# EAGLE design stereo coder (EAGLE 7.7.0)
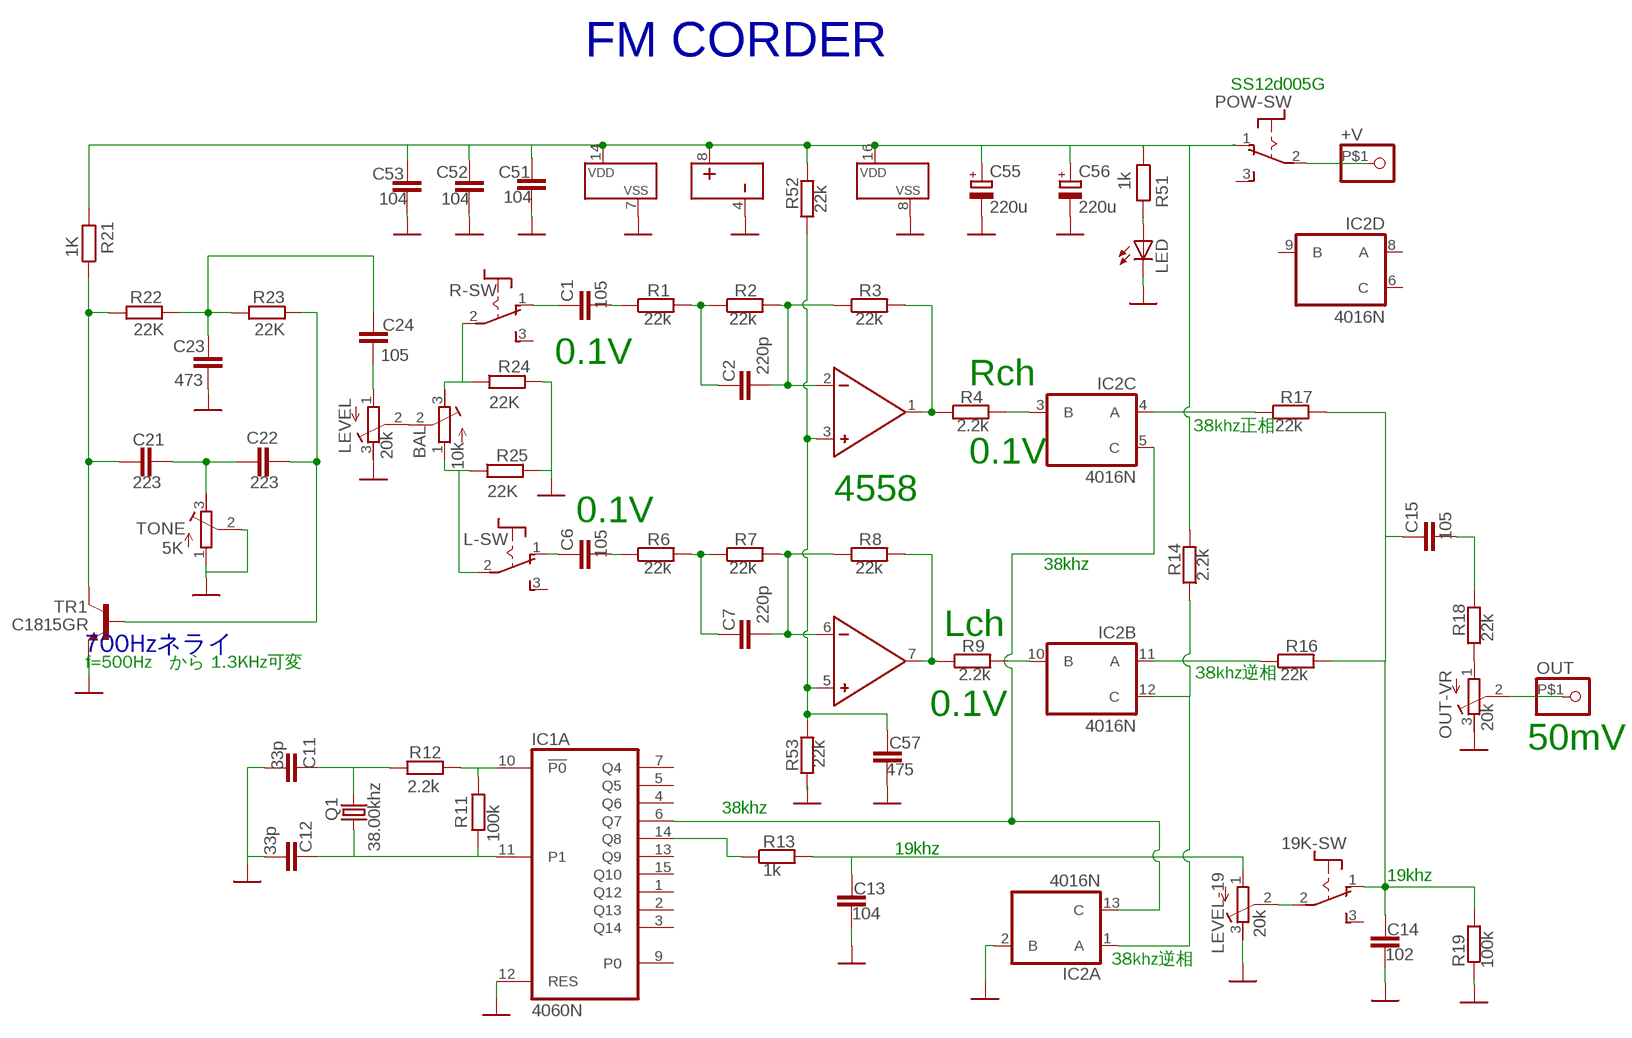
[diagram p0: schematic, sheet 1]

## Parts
19K-SW  POW-SW  [POW-SW]
+V  PINHD-1X1  [1X01]
BAL  10k  R-TRIMM3296W  [RTRIM3296W]
C1  105  C-EU050-024X044  [C050-024X044]
C2  220p  C-EU050-024X044  [C050-024X044]
C6  105  C-EU050-024X044  [C050-024X044]
C7  220p  C-EU050-024X044  [C050-024X044]
C11  33p  C-EU050-024X044  [C050-024X044]
C12  33p  C-EU050-024X044  [C050-024X044]
C13  104  C-EU050-024X044  [C050-024X044]
C14  102  C-EU050-024X044  [C050-024X044]
C15  105  C-EU050-024X044  [C050-024X044]
C21  223  C-EU050-024X044  [C050-024X044]
C22  223  C-EU050-024X044  [C050-024X044]
C23  473  C-EU050-024X044  [C050-024X044]
C24  105  C-EU050-024X044  [C050-024X044]
C51  104  C-EU050-024X044  [C050-024X044]
C52  104  C-EU050-024X044  [C050-024X044]
C53  104  C-EU050-024X044  [C050-024X044]
C55  220u  CPOL-EUE2.5-7  [E2,5-7]
C56  220u  CPOL-EUE2.5-7  [E2,5-7]
C57  475  C-EU050-024X044  [C050-024X044]
IC1  4060N  [DIL16]
IC2  4016N  [DIL14]
L-SW  POW-SW  [POW-SW]
LED  LEDIRL80A  [IRL80A]
LEVEL  20k  R-TRIMM3296W  [RTRIM3296W]
LEVEL-19  20k  R-TRIMM3296W  [RTRIM3296W]
OUT  PINHD-1X1  [1X01]
OUT-VR  20k  R-TRIMM3296W  [RTRIM3296W]
Q1  38.00khz  CRYSTALTC38H  [TC38H]
R1  22k  R-EU_0204/5  [0204/5]
R2  22k  R-EU_0204/5  [0204/5]
R3  22k  R-EU_0204/5  [0204/5]
R4  2.2k  R-EU_0204/5  [0204/5]
R6  22k  R-EU_0204/5  [0204/5]
R7  22k  R-EU_0204/5  [0204/5]
R8  22k  R-EU_0204/5  [0204/5]
R9  2.2k  R-EU_0204/5  [0204/5]
R11  100k  R-EU_0204/5  [0204/5]
R12  2.2k  R-EU_0204/5  [0204/5]
R13  1k  R-EU_0204/5  [0204/5]
R14  2.2k  R-EU_0204/5  [0204/5]
R16  22k  R-EU_0204/5  [0204/5]
R17  22k  R-EU_0204/5  [0204/5]
R18  22k  R-EU_0204/5  [0204/5]
R19  100k  R-EU_0204/5  [0204/5]
R21  1K  R-EU_0204/5  [0204/5]
R22  22K  R-EU_0204/5  [0204/5]
R23  22K  R-EU_0204/5  [0204/5]
R24  22K  R-EU_0204/5  [0204/5]
R25  22K  R-EU_0204/5  [0204/5]
R51  1k  R-EU_0204/5  [0204/5]
R52  22k  R-EU_0204/5  [0204/5]
R53  22k  R-EU_0204/5  [0204/5]
R-SW  POW-SW  [POW-SW]
TONE  5K  R-TRIMM3296W  [RTRIM3296W]
TR1  C1815GR  2SC1815L  [TO92-1815]
U$1  4558  [DIL08]
U$3  POW-SW  [POW-SW]

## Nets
+V: C51.1 C52.1 C53.1 C55.+ C56.+ IC1.16(P:VDD) IC2.14(P:VDD) R14.2 R21.2 R51.1 R52.2 U$1.8 U$3.1(O)
GND: C11.2 C12.2 C13.2 C14.2 C23.2 C51.2 C52.2 C53.2 C55.- C56.- C57.2 IC1.8(P:VSS) IC1.12(A:RES) IC2.2(A:B) IC2.7(P:VSS) LED.K(C) LEVEL-19.3(A) LEVEL.3(A) OUT-VR.3(A) R19.2 R24.2 R25.2 R53.1 TONE.1(E) TONE.2(S) TR1.E U$1.4
N$1: C2.1 R1.2 R2.1
N$2: C2.2 R2.2 R3.1 U$1.2
N$3: R3.2 R4.1 U$1.1
N$4: C1.2 R1.1
N$5: C1.1 R-SW.1(O)
N$6: C7.1 R6.2 R7.1
N$7: C7.2 R7.2 R8.1 U$1.6
N$8: R8.2 R9.1 U$1.7
N$9: C6.2 R6.1
N$10: C6.1 L-SW.1(O)
N$11: IC1.14(A:Q8) R13.1
N$13: IC2.3(C:B) R4.2
N$14: IC2.10(B:B) R9.2
N$15: IC2.4(C:A) R17.1
N$16: IC2.11(B:A) R16.1
N$17: 19K-SW.1(O) C14.1 C15.1 R16.2 R17.2 R19.1
N$18: +V.P$1 U$3.2(P)
N$19: IC1.6(A:Q7) IC2.5(C:C) IC2.13(A:C)
N$20: IC1.10(A:!P0) R11.1 R12.1
N$21: C12.1 IC1.11(A:P1) Q1.1 R11.2
N$22: C11.1 Q1.2 R12.2
N$23: C21.1 C22.2 TONE.3(A)
N$24: IC2.1(A:A) IC2.12(B:C) R14.1
N$25: C13.1 LEVEL-19.1(E) R13.2
N$26: C15.2 R18.2
N$27: C22.1 R23.2 TR1.B
N$28: C21.2 R21.1 R22.1 TR1.C
N$29: BAL.2(S) LEVEL.2(S)
N$30: LED.A R51.2
N$31: OUT-VR.1(E) R18.1
N$32: OUT-VR.2(S) OUT.P$1
N$33: 19K-SW.2(P) LEVEL-19.2(S)
N$34: C57.1 R52.1 R53.2 U$1.3 U$1.5
N$52: C23.1 C24.1 R22.2 R23.1
N$53: C24.2 LEVEL.1(E)
N$54: BAL.3(A) R24.1 R-SW.2(P)
N$55: BAL.1(E) L-SW.2(P) R25.1
Unconnected: 19K-SW.3(S) IC1.1(A:Q12) IC1.2(A:Q13) IC1.3(A:Q14) IC1.4(A:Q6) IC1.5(A:Q5) IC1.7(A:Q4) IC1.9(A:P0) IC1.13(A:Q9) IC1.15(A:Q10) IC2.6(D:C) IC2.8(D:A) IC2.9(D:B) L-SW.3(S) R-SW.3(S) U$3.3(S)

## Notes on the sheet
- FM CORDER
- SS12d005G
- 0.1V
- Rch
- 38khz正相
- 0.1V
- 4558
- 0.1V
- 38khz
- Lch
- 700Hzネライ
- f=500Hz　から 1.3KHz可変
- 38khz逆相
- 0.1V
- 50mV
- 38khz
- 19khz
- 19khz
- 38khz逆相

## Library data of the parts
19K-SW L-SW R-SW U$3 = switch:POW-SW
+V OUT = pinhead:PINHD-1X1: PIN HEADER
BAL LEVEL LEVEL-19 OUT-VR TONE = resistor:R-TRIMM: Trimm resistor
C1 C2 C6 C7 C11-C15 C21-C24 C51-C53 C57 = resistor:C-EU: CAPACITOR, European symbol
C55 C56 = resistor:CPOL-EU: POLARIZED CAPACITOR, European symbol
IC1 = 40xx:4060: 14-stage binary/ripple COUNTER
IC2 = 40xx:4016: Quad bilateral ANALOG SWITCH
LED = led:LED: LED
Q1 = crystal:CRYSTAL: CRYSTAL; OC_FARNELL: unknown; OC_NEWARK: unknown
R1-R4 R6-R9 R11-R14 R16-R19 R21-R25 R51-R53 = resistor:R-EU_: RESISTOR, European symbol
TR1 = transistor:2SC1815L
U$1 = ic-package:4558

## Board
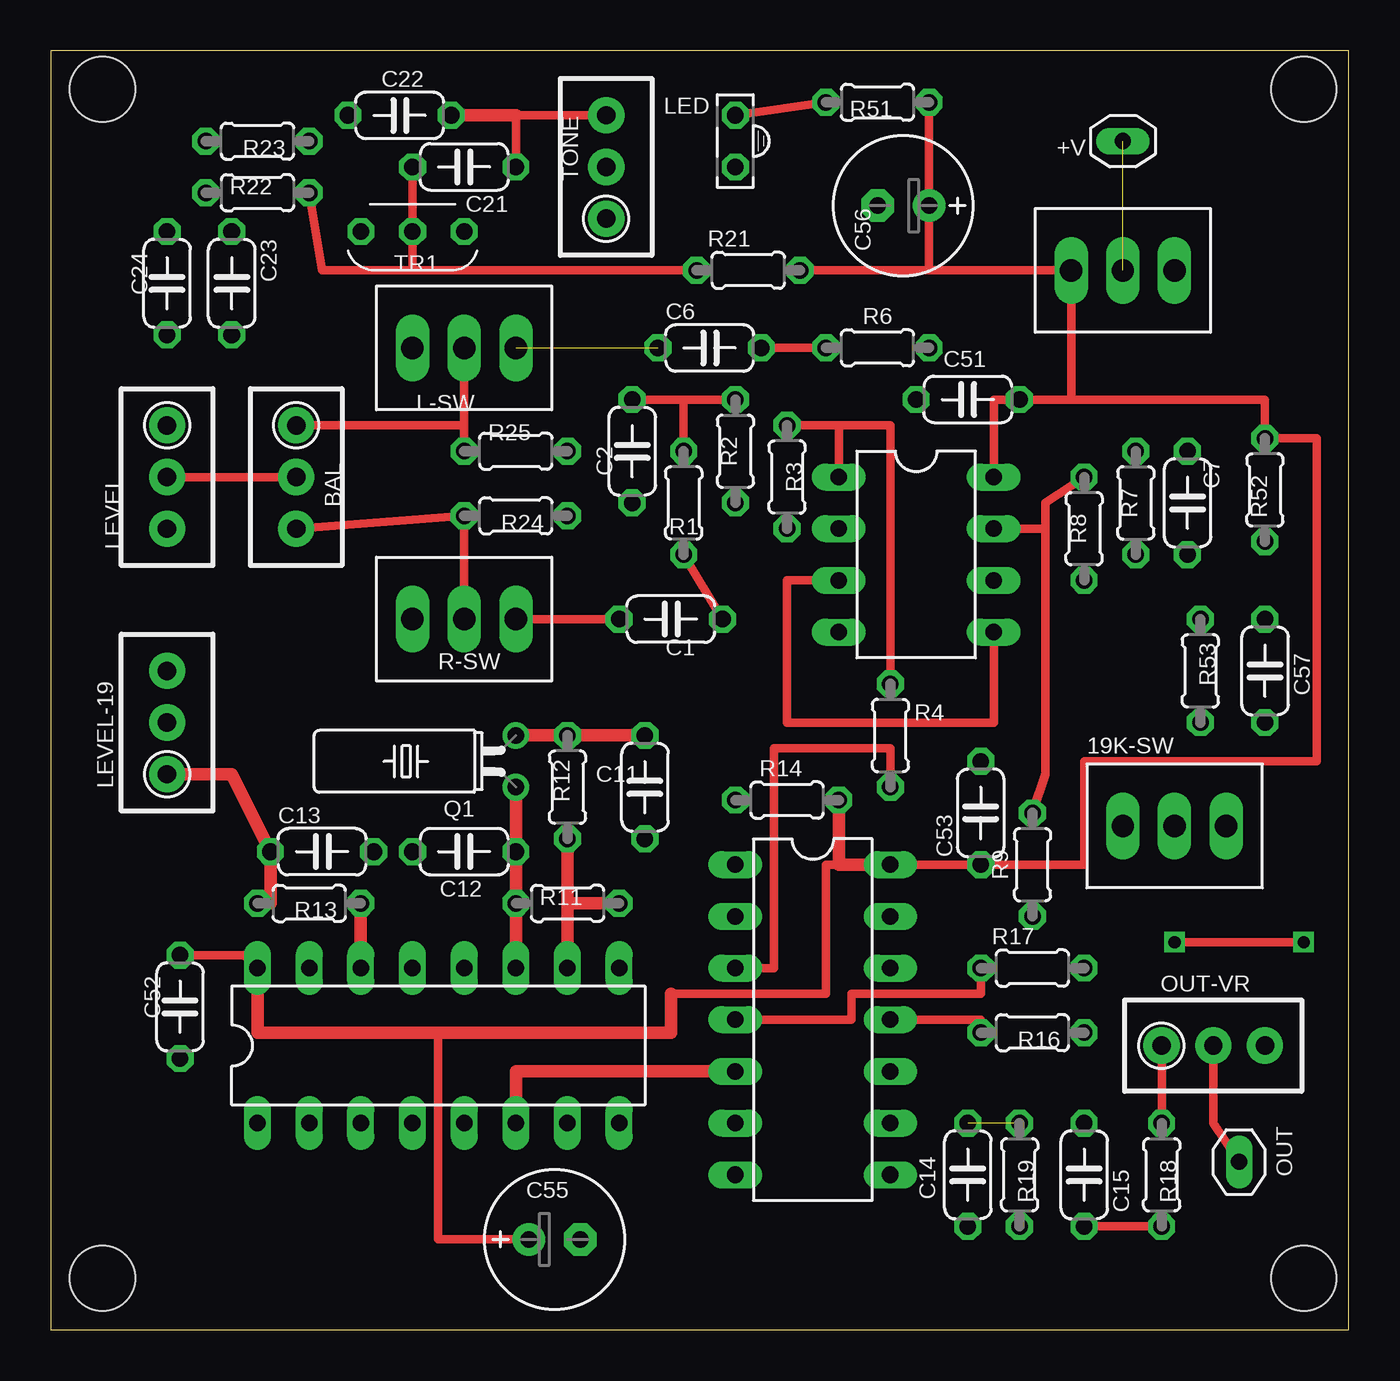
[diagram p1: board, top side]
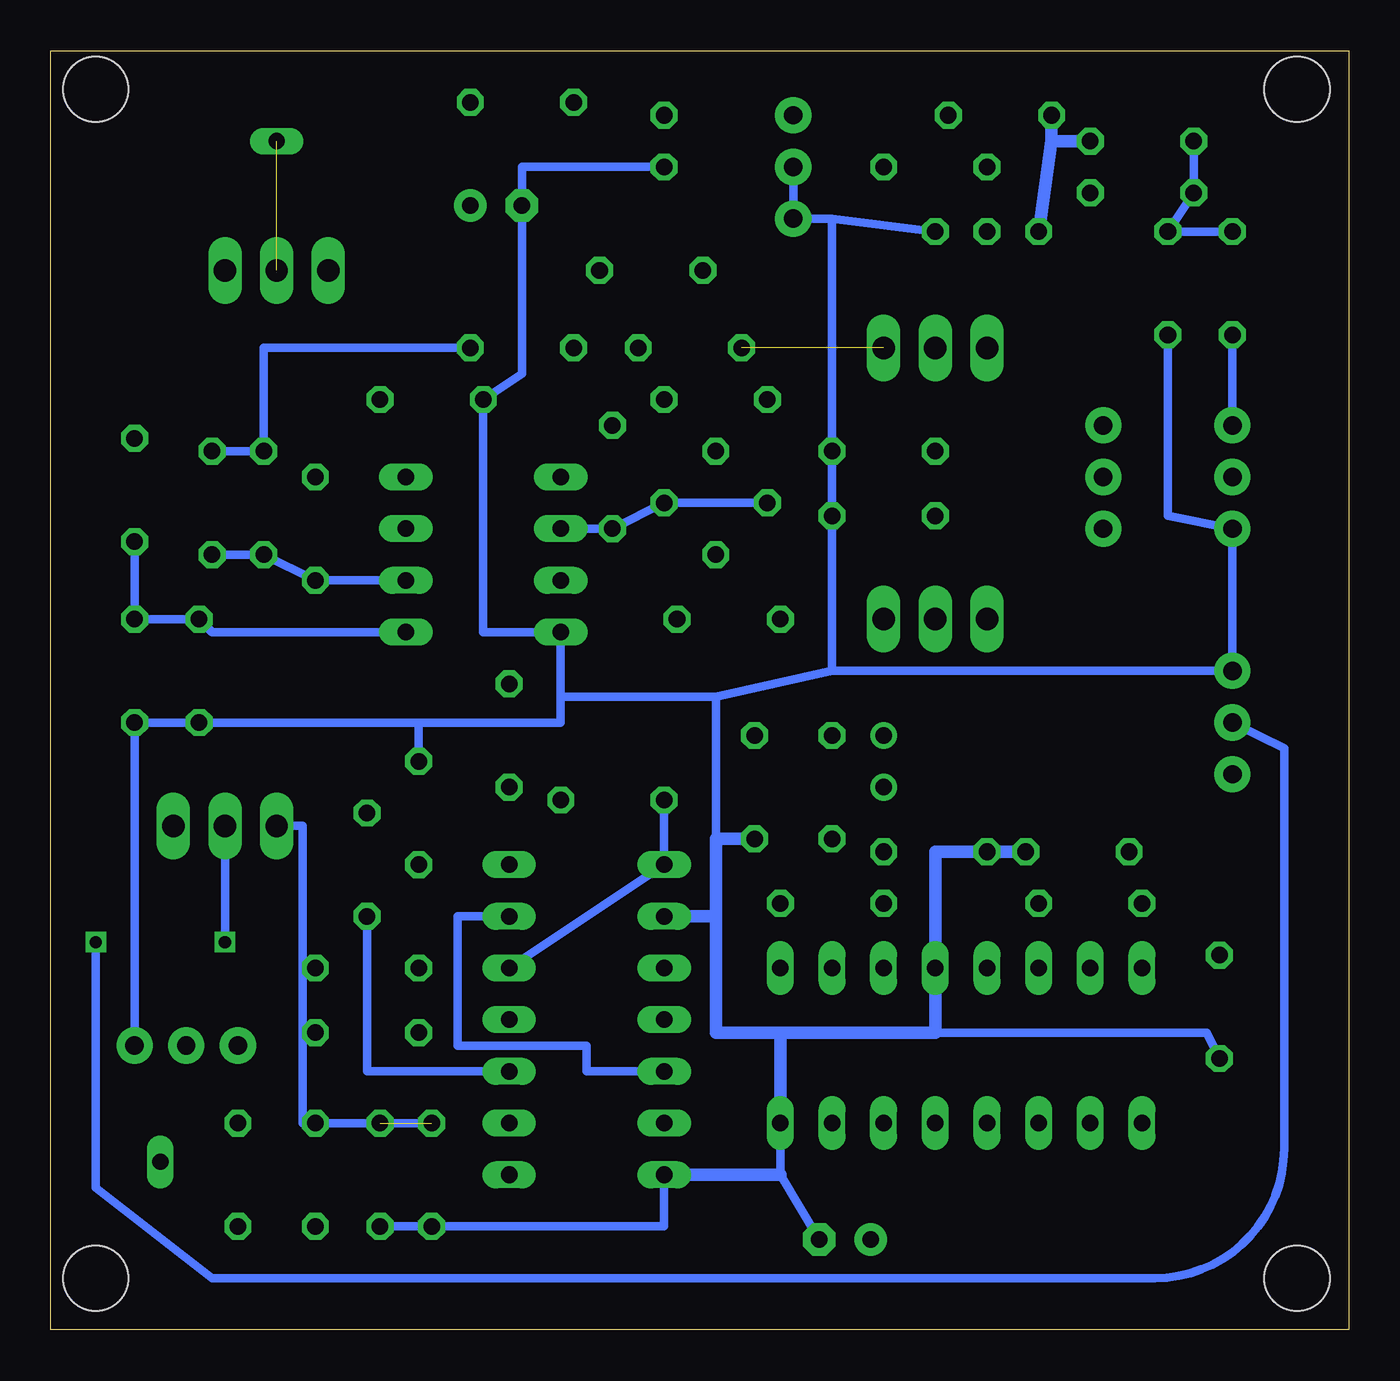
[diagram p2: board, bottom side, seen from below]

Size 63.8 x 62.86 mm. Coordinates in mm from the lower left corner, seen from the top.
Outline: 0,0 63.8,0 63.8,62.86 0,62.86 0,0
Copper layers (1*16): Top 0.035mm / dielectric 1.5mm / Bottom 0.035mm
Design rules "default": minimum track width 10mil, minimum drill 24mil, track to track 8mil, track to pad 8mil, pad to pad 8mil, via to via 8mil, smd to smd 8mil, copper to edge 40mil, drill to drill 8mil, minimum pad ring 10mil, minimum via ring 8mil, stop-mask expansion 4mil, vias tented up to drill 0mil, thermal gap 10mil
Holes 3.2 mm at 2.54,2.54 61.59,2.54 2.54,60.96 61.59,60.96

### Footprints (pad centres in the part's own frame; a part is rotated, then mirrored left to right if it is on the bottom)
POW-SW = drill 1.1 long: 1 -3.81,0; 2 -1.27,0; 3 1.27,0
1X01 = drill 0.8 long: P$1 0,0
RTRIM3296W = drill 0.9 pad 1.778: 1 0,-2.54; 2 0,0; 3 0,2.54
C050-024X044 = drill 0.813 octagon: 1 -2.54,0; 2 2.54,0
E2,5-7 = drill 0.813 pad 1.6: + -1.27,0 | drill 0.813 pad 1.6 octagon: - 1.27,0
DIL16 = drill 0.813 long: 1 -8.89,-3.81; 2 -6.35,-3.81; 3 -3.81,-3.81; 4 -1.27,-3.81; 5 1.27,-3.81; 6 3.81,-3.81; 7 6.35,-3.81; 8 8.89,-3.81; 9 8.89,3.81; 10 6.35,3.81; 11 3.81,3.81; 12 1.27,3.81; 13 -1.27,3.81; 14 -3.81,3.81; 15 -6.35,3.81; 16 -8.89,3.81
DIL14 = drill 0.813 long: 1 -7.62,-3.81; 2 -5.08,-3.81; 3 -2.54,-3.81; 4 0,-3.81; 5 2.54,-3.81; 6 5.08,-3.81; 7 7.62,-3.81; 8 7.62,3.81; 9 5.08,3.81; 10 2.54,3.81; 11 0,3.81; 12 -2.54,3.81; 13 -5.08,3.81; 14 -7.62,3.81
IRL80A = drill 0.813 octagon: A 0,-1.27; K 0,1.27
TC38H = drill 0.813: 1 -1.27,0; 2 1.27,0
0204/5 = drill 0.813 octagon: 1 -2.54,0; 2 2.54,0
TO92-1815 = drill 0.813 octagon: B 2.54,0; C 0,0; E -2.54,0
DIL08 = drill 0.813 long: 1 -3.81,-3.81; 2 -1.27,-3.81; 3 1.27,-3.81; 4 3.81,-3.81; 5 3.81,3.81; 6 1.27,3.81; 7 -1.27,3.81; 8 -3.81,3.81

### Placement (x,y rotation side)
19K-SW  56.52,24.77 0 top
+V  52.7,58.42 0 top
BAL  12.07,41.91 180 top
C1  30.48,34.92 0 top
C2  28.57,43.18 270 top
C6  32.39,48.26 0 top
C7  55.88,40.64 270 top
C11  29.21,26.67 270 top
C12  20.32,23.49 180 top
C13  13.34,23.49 0 top
C14  45.08,7.62 270 top
C15  50.8,7.62 270 top
C21  20.32,57.15 180 top
C22  17.14,59.69 0 top
C23  8.89,51.44 270 top
C24  5.71,51.44 270 top
C51  45.08,45.72 180 top
C52  6.35,15.88 270 top
C53  45.72,25.4 90 top
C55  24.76,4.44 0 top
C56  41.91,55.24 180 top
C57  59.69,32.38 270 top
IC1  19.05,13.97 0 top
IC2  37.47,15.24 270 top
L-SW  19.05,48.26 180 top
LED  33.66,58.42 180 top
LEVEL  5.71,41.91 180 top
LEVEL-19  5.71,29.84 0 top
OUT  58.42,8.26 90 top
OUT-VR  57.15,13.97 270 top
Q1  22.86,27.94 90 top
R1  31.11,40.64 90 top
R2  33.66,43.18 270 top
R3  36.19,41.91 90 top
R4  41.28,29.21 270 top
R6  40.64,48.26 0 top
R7  53.34,40.64 270 top
R8  50.8,39.37 90 top
R9  48.26,22.86 270 top
R11  25.4,20.95 180 top
R12  25.4,26.67 90 top
R13  12.7,20.95 180 top
R14  36.19,26.04 0 top
R16  48.26,14.61 0 top
R17  48.26,17.78 0 top
R18  54.61,7.62 270 top
R19  47.62,7.62 270 top
R21  34.29,52.07 0 top
R22  10.16,55.88 180 top
R23  10.16,58.42 0 top
R24  22.86,40 0 top
R25  22.86,43.18 0 top
R51  40.64,60.32 180 top
R52  59.69,41.27 90 top
R53  56.52,32.38 90 top
R-SW  19.05,34.92 180 top
TONE  27.3,57.15 0 top
TR1  17.78,53.98 180 top
U$1  42.55,38.1 270 top
U$3  53.97,52.07 0 top

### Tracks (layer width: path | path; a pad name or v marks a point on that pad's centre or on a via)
+V
  Top 0.406: 30.48,16.51 38.1,16.51 38.1,22.86 38.73,22.86 | C55.+ 19.05,4.44 19.05,14.61 | 50.16,45.72 C51.1 46.36,45.72 U$1.8 | 50.16,45.72 59.69,45.72 R52.2 62.23,43.81 62.23,27.94 50.8,27.94 50.8,22.86 C53.1 IC2.14 | C52.1 9.52,18.41 IC1.16 | 50.16,45.72 U$3.1 43.18,52.07 | 43.18,52.07 R21.2 | R51.1 C56.+ 43.18,52.07
  Top 0.61: IC1.16 10.16,14.61 19.05,14.61 30.48,14.61 30.48,16.51 | R14.2 38.73,22.86 IC2.14
GND
  Bottom 0.406: 31.11,31.12 31.11,24.13 | IC1.8 27.94,7.62 C55.- | OUT-VR.3 C57.2 R53.1 45.72,29.84 | 38.73,31.12 U$1.4 42.55,34.29 C51.2 40.64,46.99 C56.- 40.64,57.15 LED.K | 38.73,31.12 38.73,29.84 45.72,29.84 | 25.4,32.38 R24.2 R25.2 25.4,54.61 | 25.4,54.61 TR1.E | C23.2 8.89,40 LEVEL.3 LEVEL-19.3 25.4,32.38 | 25.4,32.38 31.11,31.12 | IC2.7 33.66,5.08 C14.2 R19.2 | C53.2 45.72,29.84 | 20.32,14.61 6.98,14.61 C52.2 | 31.11,31.12 38.73,31.12 | TONE.2 TONE.1 25.4,54.61
  Bottom 0.61: 27.94,14.61 20.32,14.61 IC1.12 20.32,23.49 C12.2 C13.2 | 27.94,14.61 IC1.8 | C11.2 31.11,24.13 31.11,20.32 | 31.11,20.32 31.11,14.61 27.94,14.61 | IC2.7 27.94,7.62 | IC2.2 31.11,20.32
N$1
  Top 0.406: R2.1 31.11,45.72 | 31.11,45.72 C2.1 | R1.2 31.11,45.72
N$2
  Bottom 0.406: C2.2 R2.2 R3.1 U$1.2
N$3
  Top 0.406: R3.2 38.73,44.45 | 38.73,44.45 41.28,44.45 R4.1 | U$1.1 38.73,44.45
N$4
  Top 0.406: C1.2 R1.1
N$5
  Top 0.406: R-SW.1 C1.1
N$6
  Bottom 0.406: R6.2 53.34,48.26 R7.1 C7.1
N$7
  Bottom 0.406: U$1.6 R8.1 R7.2 C7.2
N$8
  Top 0.406: U$1.7 48.89,39.37 | R8.2 48.89,40.64 48.89,39.37 | 48.89,39.37 48.89,27.3 R9.1
N$9
  Top 0.406: R6.1 C6.2
N$10  (1 unrouted)
N$11
  Top 0.61: R13.1 IC1.14
N$13
  Top 0.406: IC2.3 35.56,17.78 35.56,28.57 41.28,28.57 R4.2
N$14
  Bottom 0.406: R9.2 48.26,12.7 IC2.10
N$15
  Top 0.406: IC2.4 39.37,15.24 39.37,16.51 45.72,16.51 R17.1
N$16
  Top 0.406: IC2.11 45.72,15.24 R16.1
N$17  (1 unrouted)
  Bottom 0.406: R17.2 51.44,17.78 | 51.44,17.78 51.44,14.61 | 51.44,14.61 R16.2 | 51.44,14.61 51.44,10.16 C15.1 C14.1 | 19K-SW.1 51.44,24.77 51.44,17.78
N$18  (1 unrouted)
N$19
  Top 0.61: IC1.6 22.86,12.7 IC2.5
  Bottom 0.406: IC2.5 37.47,12.7 37.47,13.97 43.81,13.97 43.81,20.32 IC2.13
N$20
  Top 0.61: R12.1 25.4,20.95 | 25.4,20.95 IC1.10 | R11.1 25.4,20.95
N$21
  Top 0.61: Q1.1 C12.1 R11.2 IC1.11
N$22
  Top 0.61: Q1.2 R12.2 C11.1
N$23
  Top 0.406: TONE.3 22.86,59.69 C21.1
  Top 0.61: C22.2 22.86,59.69
N$24
  Bottom 0.406: R14.1 IC2.1 IC2.12
N$25
  Top 0.61: LEVEL-19.1 8.89,27.3 C13.1 10.79,20.95 R13.2
N$26
  Top 0.406: C15.2 R18.2
N$27
  Bottom 0.61: TR1.B 14.61,58.42 | 14.61,58.42 R23.2 | C22.1 14.61,58.42
N$28
  Top 0.406: 17.78,52.07 TR1.C C21.2 | 17.78,52.07 R21.1 | R22.1 13.34,52.07 17.78,52.07
N$29
  Top 0.406: LEVEL.2 BAL.2
N$30
  Top 0.406: R51.2 LED.A
N$31
  Top 0.406: OUT-VR.1 R18.1
N$32
  Top 0.406: OUT-VR.2 57.15,10.16 OUT.P$1
N$33  (via drill 0.6)
  Top 0.406: v61.59,19.05 v55.24,19.05
  Bottom 0.406: LEVEL-19.2 3.18,28.57 3.18,8.89 arc90 9.52,2.54 55.88,2.54 61.59,6.99 v61.59,19.05 | v55.24,19.05 19K-SW.2
N$34
  Top 0.406: U$1.3 36.19,36.83 36.19,29.84 46.36,29.84 U$1.5
  Bottom 0.406: U$1.5 55.88,34.29 R53.2 C57.1 R52.1
N$52
  Bottom 0.406: R23.1 R22.2 C23.1 C24.1
N$53
  Bottom 0.406: C24.2 LEVEL.1
N$54
  Top 0.406: BAL.3 R24.1 R-SW.2
N$55
  Top 0.406: BAL.1 20.32,44.45 | 20.32,44.45 R25.1 | L-SW.2 20.32,44.45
